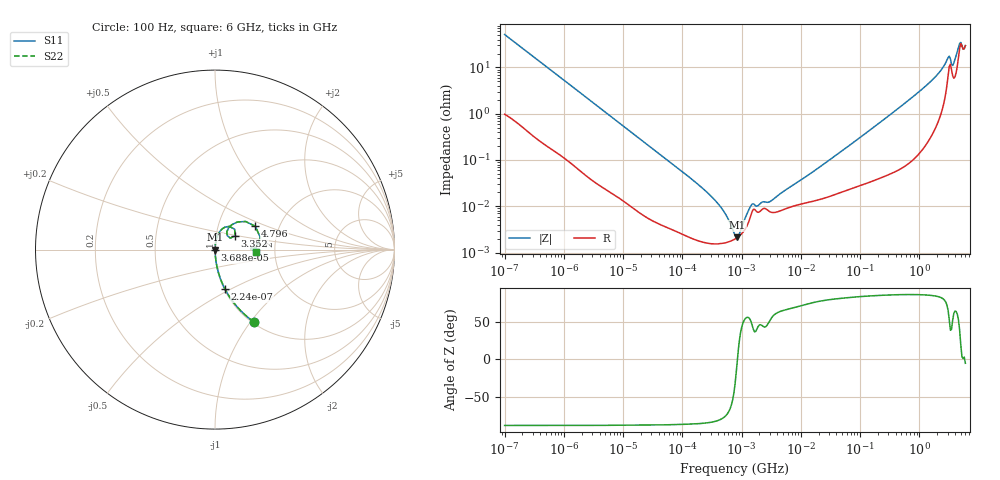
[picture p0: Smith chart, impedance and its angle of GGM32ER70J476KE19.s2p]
!Murata Part Number: GGM32ER70J476KE19
!These Parameters are Measured in Series Mode Connection
!Data Generated on Jun 19, 2026
!  o--ll--o
!Port1  Port2
!  o------o
!Operation Temp=25[degC], DC Bias Voltage=0[V]
!Freq. Start=100[Hz] Stop=6[GHz] 401[Steps]
# Hz S RI R 50
!Freq.(Hz) S11(Real) S11(Imag) S21(Real) S21(Imag) S12(Real) S12(Imag) S22(Real) S22(Imag)
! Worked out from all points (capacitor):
!   401 points, 100 Hz to 6 GHz, reference 50 ohm
!   read as one part in series: C = 30.6 uF near 109 Hz
!   lowest |Z| = 2.12 mohm at 847.2 kHz (marker M1)
!   series resonance near 850.2 kHz, so ESL is about 1.1 nH
!   S11 on the Smith chart (normalised r, x): 100 Hz: 1.02, -1.03; 224 Hz: 1.01, -0.47; 36.88 kHz: 1.00, -0.00; 3.352 GHz: 1.24, +0.19; 4.796 GHz: 1.51, +0.42; 6 GHz: 1.59, -0.05
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100  0.2155 -0.4019  0.7845 0.4019  0.7845 0.4019  0.2155 -0.4019
224  0.0557 -0.2199  0.9443 0.2199  0.9443 0.2199  0.0557 -0.2199
573  0.0102 -0.0912  0.9898 0.0912  0.9898 0.0912  0.0102 -0.0912
2008  0.00126 -0.0268  0.9987 0.0268  0.9987 0.0268  0.00126 -0.0268
36880  4.6e-05 -0.00151  1 0.00151  1 0.00151  4.6e-05 -0.00151
40335  4.34e-05 -0.00138  1 0.00138  1 0.00138  4.34e-05 -0.00138
184852  1.81e-05 -0.000296  1 0.000296  1 0.000296  1.81e-05 -0.000296
432798  1.56e-05 -9.97e-05  1 9.97e-05  1 9.97e-05  1.56e-05 -9.97e-05
774597  1.97e-05 -1.31e-05  1 1.31e-05  1 1.31e-05  1.97e-05 -1.31e-05
847162  2.12e-05 -5e-07  1 5e-07  1 5e-07  2.12e-05 -5e-07
1813585  7.59e-05 6.61e-05  0.9999 -6.61e-05  0.9999 -6.61e-05  7.59e-05 6.61e-05
2967816  7.71e-05 9.84e-05  0.9999 -9.84e-05  0.9999 -9.84e-05  7.71e-05 9.84e-05
1.555665e7  0.000128 0.000527  0.9999 -0.000527  0.9999 -0.000527  0.000128 0.000527
3.124326e8  0.000575 0.00925  0.9994 -0.00925  0.9994 -0.00925  0.000575 0.00925
1.565993e9  0.00562 0.0498  0.9944 -0.0498  0.9944 -0.0498  0.00562 0.0498
2.240541e9  0.015 0.0798  0.985 -0.0798  0.985 -0.0798  0.015 0.0798
2.931063e9  0.0566 0.1255  0.9434 -0.1255  0.9434 -0.1255  0.0566 0.1255
3.352442e9  0.1125 0.0771  0.8875 -0.0771  0.8875 -0.0771  0.1125 0.0771
3.8344e9  0.0657 0.0982  0.9343 -0.0982  0.9343 -0.0982  0.0657 0.0982
4.385646e9  0.1244 0.1537  0.8756 -0.1537  0.8756 -0.1537  0.1244 0.1537
4.796499e9  0.2247 0.13  0.7753 -0.13  0.7753 -0.13  0.2247 0.13
6e9  0.2288 -0.0156  0.7712 0.0156  0.7712 0.0156  0.2288 -0.0156
